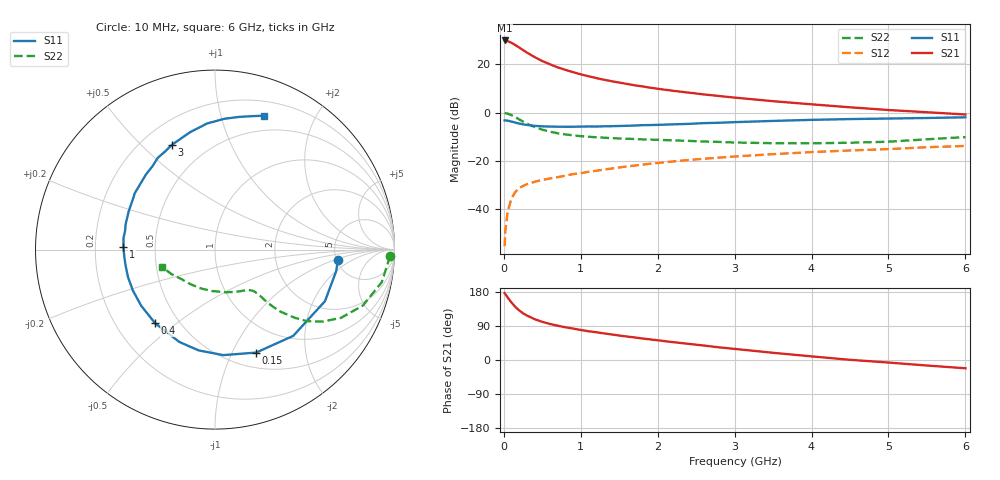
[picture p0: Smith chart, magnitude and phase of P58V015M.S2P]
! SIEMENS Small Signal Semiconductors
! BFP183
! Si NPN RF Bipolar Junction Transistor in SOT143
! VCE = 8 V  IC = 15 mA
! Common Emitter S-Parameters:  March  1996
# GHz  S  MA  R  50
!  f  S11  S21  S12  S22
! GHz  MAG  ANG  MAG  ANG  MAG  ANG  MAG  ANG
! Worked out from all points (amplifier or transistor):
!   36 points, 10 MHz to 6 GHz, reference 50 ohm
!   highest |S21| = 29.9 dB at 10 MHz (marker M1)
!   |S21| within 3 dB of that: start of sweep to 202.9 MHz
!   unconditionally stable (mu >= 1): 1.105 GHz to 5.798 GHz
!   at 250 MHz: K = 0.38, MSG = 28.1 dB, |S12| = -30.4 dB
!   at 1.4 GHz: K = 1.08, MAG = 16.4 dB, |S12| = -23.2 dB
!   at 6 GHz: K = 0.98, MSG = 6.5 dB, |S12| = -13.9 dB
!   S11 on the Smith chart (normalised r, x): 10 MHz: 5.14, -1.12; 150 MHz: 0.67, -1.24; 400 MHz: 0.37, -0.42; 1 GHz: 0.32, +0.01; 3 GHz: 0.32, +0.62; 6 GHz: 0.34, +1.38
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0.01  0.687 -4.8  31.1 176.4  0.0017 75.0  0.9743 -2.1
0.02  0.6861 -9.9  31.06 173.9  0.0036 83.7  0.9664 -4.4
0.05  0.6768 -25.1  30.19 164.9  0.0089 79.8  0.9471 -11.0
0.1  0.6488 -47.8  27.71 151.6  0.0166 67.7  0.881 -20.7
0.15  0.6179 -68.2  24.96 140.0  0.0227 60.7  0.7989 -28.4
0.2  0.5897 -85.5  22.17 130.7  0.0271 56.1  0.7197 -33.9
0.25  0.569 -99.1  19.58 123.1  0.0301 51.5  0.6489 -37.9
0.3  0.5517 -111.1  17.47 117.4  0.0327 49.3  0.588 -40.4
0.4  0.5288 -129.1  14.07 107.7  0.0366 46.9  0.5011 -43.5
0.5  0.5167 -142.7  11.63 100.7  0.0401 45.4  0.4412 -44.8
0.6  0.5111 -153.7  9.987 95.1  0.043 45.1  0.4007 -45.4
0.7  0.5083 -162.4  8.604 90.5  0.0458 46.2  0.3714 -45.6
0.8  0.506 -169.5  7.649 86.3  0.049 46.2  0.3513 -45.8
1  0.5103 178.3  6.169 79.3  0.0552 47.3  0.3237 -46.6
1.1  0.5137 172.8  5.648 75.9  0.0592 47.5  0.3143 -47.2
1.5  0.5258 156.2  4.167 64.5  0.0726 47.8  0.2899 -51.0
2.2  0.5684 132.6  2.817 47.1  0.0968 44.7  0.264 -62.3
3  0.6317 112.2  2.036 29.3  0.1225 39.0  0.2388 -80.5
3.5  0.669 101.9  1.716 19.0  0.1371 35.1  0.2313 -94.2
4.5  0.7308 85.9  1.282 0.5  0.1635 26.9  0.2363 -125.2
5.5  0.7694 75.0  1.013 -14.6  0.1908 19.8  0.2786 -150.7
6  0.795 69.8  0.909 -21.8  0.2027 15.3  0.3096 -161.7
